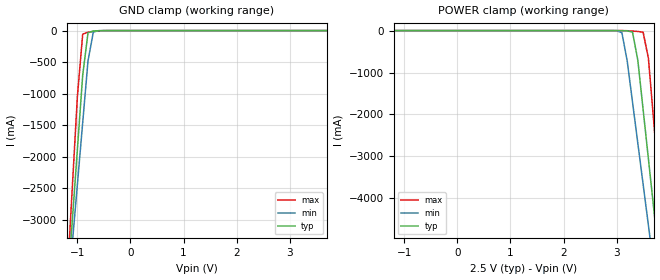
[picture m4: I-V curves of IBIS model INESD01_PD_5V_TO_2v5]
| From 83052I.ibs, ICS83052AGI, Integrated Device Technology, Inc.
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[Model] INESD01_PD_5V_TO_2v5
Model_type   Input
Polarity   Non-Inverting
Vinl = 0.8V
Vinh = 2.0V
|   typ   min   max
C_comp   2pF   1.5pF   2.5pF
|   typ   min   max
[Voltage range]  2.5V   2.375V   2.625V
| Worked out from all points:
|   GND clamp passes 1 mA (typ) near -0.54 V on its own axis
[GND_clamp]
|Voltage I(typ)   I(min)   I(max)
-2.5V     -19.6A     -17.18A    -23.67A
-1.2V     -4.246A    -4.402A    -4.061A
-1.1V     -3.066A    -3.421A    -2.553A
-1V       -1.886A    -2.44A     -1.044A
-900mV    -707.1mA   -1.46A     -57.39mA
-800mV    -35.57mA   -480.7mA   -24.35mA
-700mV    -6.978mA   -23.99mA   -13.24mA
-600mV    -2.058mA   -1.658mA   -4.859mA
-500mV    -351.6uA   -178.6uA   -861.9uA
5V        97.41uA    121.8uA    92.26uA
[POWER_clamp]
|Voltage   I(typ)   I(min)   I(max)
-2.5V     97.41uA    118.8uA    94.56uA
2.9V      -40.75uA   -304.9uA   -6.154uA
3.1V      -2.058mA   -50.97mA   -496.5uA
3.2V      -6.978mA   -725.3mA   -3.411mA
3.3V      -35.57mA   -1.704A    -10.82mA
3.4V      -707.1mA   -2.685A    -21.35mA
3.5V      -1.886A    -3.666A    -39.37mA
3.6V      -3.066A    -4.647A    -666.9mA
3.7V      -4.246A    -5.629A    -2.175A
3.8V      -5.426A    -6.612A    -3.684A
3.9V      -6.607A    -7.594A    -5.193A
5V        -19.6A     -18.41A    -21.79A
